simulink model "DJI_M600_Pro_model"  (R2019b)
settings: Solver=FixedStepAuto  StartTime=0.0  StopTime=stop_time  FixedStep=ts_hexacopter  RelTol=1e-3
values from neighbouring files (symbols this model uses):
  Alt_den = [0.1 1 0]    [Model_3D_init.m]
  Alt_err = 0.3817    [Model_3D_init.m]
  Alt_num = -[2 1]*18    [Model_3D_init.m]
  DvD = -5    [Model_3D_init.m]
  DvN = -17    [Model_3D_init.m]
  DvT = -17    [Model_3D_init.m]
  flightctrl_flag = bin2dec([HorizontalLogic; VerticalLogic; YawLogic; HorizontalCoordinate; StableMode]')    [User_defined_3D_init_run.m]
  Pden = [0.01 1]    [Model_3D_init.m]
  PI = -0.03    [Model_3D_init.m]
  pitch_max = 25/180*pi    (= 0.436332312999)    [Model_3D_init.m]
  Pnum = 100*[0.25 5]    [Model_3D_init.m]
  PP = -0.07    [Model_3D_init.m]
  r_max = 2.618    [Model_3D_init.m]
  r_min = -2.618    [Model_3D_init.m]
  Rden = [0.01 1]    [Model_3D_init.m]
  RI = 0.03    [Model_3D_init.m]
  Rnum = 100*[0.32 5]    [Model_3D_init.m]
  roll_max = 25/180*pi    (= 0.436332312999)    [Model_3D_init.m]
  RP = 0.07    [Model_3D_init.m]
  ts_hexacopter = 0.005    [Model_3D_init.m]
  UvD = 5    [Model_3D_init.m]
  UvN = 17    [Model_3D_init.m]
  UvT = 17    [Model_3D_init.m]
  Xtype = 3    [User_defined_3D_init_run.m]
  Yaw_den = [ET 1 0]    [Model_3D_init.m]
  Yaw_num = Eg*[1 Ez]    [Model_3D_init.m]
  YAWtype = 1    [User_defined_3D_init_run.m]
  Ytype = 1    [User_defined_3D_init_run.m]
  Ztype = 1    [User_defined_3D_init_run.m]
undefined symbols (not defined in the file or in its folder): DiscIntNeverNeededParam, params, Xdoublet, Xstep, YAWdoublet, YAWstep, Ydoublet, Ystep, Zdoublet, Zstep
libraries: simulink x1
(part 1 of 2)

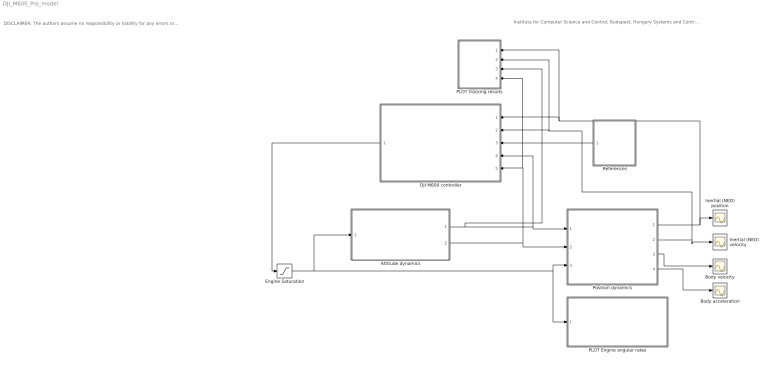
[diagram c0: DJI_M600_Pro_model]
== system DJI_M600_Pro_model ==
  note: Institute for Computer Science and Control, Budapest, Hungary Systems and Control Laboratory 2023. v3.0 12. June 2023. NED ground coordinate system and aligned (X forward, Y right, Z down) body system are applied
  note: DISCLAIMER: The authors assume no responsibility or liability for any errors or omissions in this model and any errors or damages (including loss of property or life) caused by the use of this model . The model is provided on an "as is" basis with no guarantees of fitting any specific need or goal. Application of the model in flight control design or in any application of a DJI M600 hexacopter is solely the responsibility of the user.
  Attitude dynamics : Subsystem
  Body acceleration : Scope
  Body velocity : Scope
  DJI M600 controller : Subsystem
  Engine Saturation : Saturate  UpperLimit=params.engine_saturation  LowerLimit=0
  Inertial (NED) position : Scope
  Inertial (NED) velocity : Scope
  PLOT Engine angular rates : Subsystem
  PLOT tracking results : Subsystem
  Position dynamics : Subsystem
  References : Subsystem
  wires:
  Position dynamics/1(position) -> Inertial (NED) position/1, DJI M600 controller/1(NED position), PLOT tracking results/1(NED position)
  Position dynamics/2(v_I) -> DJI M600 controller/2(NED velocity), PLOT tracking results/2(NED velocity), Inertial (NED) velocity/1
  Position dynamics/3(v_B) -> Body velocity/1
  Position dynamics/4(a_B) -> Body acceleration/1
  DJI M600 controller/1(Engine_Om_CTRL) -> Engine Saturation/1
  References/1(References) -> DJI M600 controller/3(References)
  Attitude dynamics/1(Euler angles) -> Position dynamics/1(Euler angles), DJI M600 controller/4(Euler angles), PLOT tracking results/3(Euler angles)
  Attitude dynamics/2(Omega_B) -> PLOT tracking results/4(Angular rates), DJI M600 controller/5(Angular rates), Position dynamics/2(Angular velocities)
  Engine Saturation/1 -> Attitude dynamics/1(Omega engine angualr), Position dynamics/3(Omega engine angular), PLOT Engine angular rates/1(Engine angular rates)

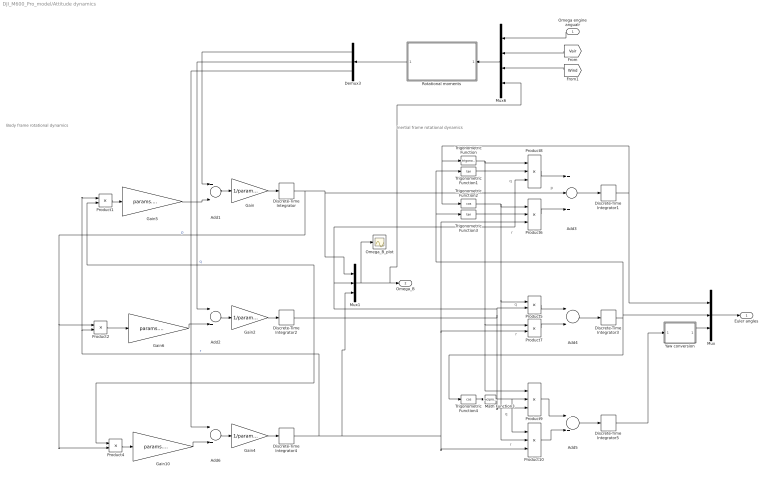
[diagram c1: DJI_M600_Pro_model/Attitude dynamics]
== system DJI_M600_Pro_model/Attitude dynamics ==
  note: r
  note: q
  note: r
  note: q
  note: r
  note: q
  note: p
  note: Inertial frame rotational dynamics
  note: Body frame rotational dynamics
  Omega engine angualr : Inport
  Add{1..2,5..6} (4 alike) : Sum
  Add3 : Sum  Inputs=+++
  Add4 : Sum  Inputs=+-
  Demux3 : Demux  Outputs=[1; 1; 1]
  Discrete-Time Integrator : DiscreteIntegrator  InitialCondition=params.initial_angvel(1)  SampleTime=ts_hexacopter  ICPrevOutput=DiscIntNeverNeededParam  ICPrevScaledInput=DiscIntNeverNeededParam
  Discrete-Time Integrator1 : DiscreteIntegrator  InitialCondition=params.initial_euler(1)  SampleTime=ts_hexacopter  ICPrevOutput=DiscIntNeverNeededParam  ICPrevScaledInput=DiscIntNeverNeededParam
  Discrete-Time Integrator2 : DiscreteIntegrator  InitialCondition=params.initial_angvel(2)  SampleTime=ts_hexacopter  ICPrevOutput=DiscIntNeverNeededParam  ICPrevScaledInput=DiscIntNeverNeededParam
  Discrete-Time Integrator3 : DiscreteIntegrator  InitialCondition=params.initial_euler(2)  SampleTime=ts_hexacopter  ICPrevOutput=DiscIntNeverNeededParam  ICPrevScaledInput=DiscIntNeverNeededParam
  Discrete-Time Integrator4 : DiscreteIntegrator  InitialCondition=params.initial_angvel(3)  SampleTime=ts_hexacopter  ICPrevOutput=DiscIntNeverNeededParam  ICPrevScaledInput=DiscIntNeverNeededParam
  Discrete-Time Integrator5 : DiscreteIntegrator  InitialCondition=params.initial_euler(3)  SampleTime=ts_hexacopter  ICPrevOutput=DiscIntNeverNeededParam  ICPrevScaledInput=DiscIntNeverNeededParam
  Gain : Gain  Gain=1/params.Jxx
  Gain10 : Gain  Gain=params.Jxx-params.Jyy
  Gain2 : Gain  Gain=1/params.Jyy
  Gain4 : Gain  Gain=1/params.Jzz
  Gain5 : Gain  Gain=params.Jyy-params.Jzz
  Gain6 : Gain  Gain=params.Jzz-params.Jxx
  Math Function3 : Math  Operator=reciprocal
  Mux : Mux  Inputs=[1; 1; 1]
  Mux1 : Mux  Inputs=[1; 1; 1]
  Mux6 : Mux  Inputs=[6; 3; 3; 3]
  Omega_B_plot : Scope
  Product{1..2,4..5,7} (5 alike) : Product
  Product{6,8..10} (4 alike) : Product  Inputs=3
  Rotational moments : MATLAB Function  TreatAsAtomicUnit=on
  Trigonometric Function : Trigonometry
  Trigonometric Function1 : Trigonometry  Operator=tan
  Trigonometric Function2 : Trigonometry  Operator=cos
  Trigonometric Function3 : Trigonometry  Operator=tan
  Trigonometric Function4 : Trigonometry  Operator=cos
  Yaw conversion : MATLAB Function  TreatAsAtomicUnit=on  SystemSampleTime=ts_hexacopter
  Euler angles : Outport
  Omega_B : Outport  Port=2
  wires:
  Gain/1 -> Discrete-Time Integrator/1
  Add1/1 -> Gain/1
  Discrete-Time Integrator/1 -> Product4/2, Product2/1, Mux1/1, Add3/2  "p"
  Discrete-Time Integrator1/1 -> Trigonometric Function2/1, Trigonometric Function/1, Mux/1
  Discrete-Time Integrator2/1 -> Product4/1, Product1/2, Product9/3, Mux1/2, Product8/3, Product5/2  "q"
  Discrete-Time Integrator3/1 -> Trigonometric Function3/1, Trigonometric Function1/1, Mux/2, Trigonometric Function4/1
  Gain2/1 -> Discrete-Time Integrator2/1
  Discrete-Time Integrator4/1 -> Product2/2, Product1/1, Mux1/3, Product10/3, Product7/2, Product6/3  "r"
  Gain4/1 -> Discrete-Time Integrator4/1
  Discrete-Time Integrator5/1 -> Yaw conversion/1(u)
  Product1/1 -> Gain5/1
  Product2/1 -> Gain6/1
  Product4/1 -> Gain10/1
  Add3/1 -> Discrete-Time Integrator1/1
  Trigonometric Function/1 -> Product9/1, Product7/1, Product8/1
  Trigonometric Function1/1 -> Product8/2
  Trigonometric Function2/1 -> Product10/2, Product5/1, Product6/1
  Trigonometric Function3/1 -> Product6/2
  Product6/1 -> Add3/3
  Product8/1 -> Add3/1
  Add4/1 -> Discrete-Time Integrator3/1
  Product5/1 -> Add4/1
  Product7/1 -> Add4/2
  Add5/1 -> Discrete-Time Integrator5/1
  Product9/1 -> Add5/1
  Product10/1 -> Add5/2
  Trigonometric Function4/1 -> Math Function3/1
  Math Function3/1 -> Product10/1, Product9/2
  Mux1/1 -> Omega_B_plot/1, Mux6/4, Omega_B/1
  Gain5/1 -> Add1/2
  Add2/1 -> Gain2/1
  Add6/1 -> Gain4/1
  Gain10/1 -> Add6/2
  Gain6/1 -> Add2/2
  Rotational moments/1(y) -> Demux3/1
  Mux6/1 -> Rotational moments/1(u)
  Demux3/1 -> Add1/1
  Demux3/2 -> Add2/1
  Demux3/3 -> Add6/1
  Omega engine angualr/1 -> Mux6/1
  [Vair] -> Mux6/2
  [Wind] -> Mux6/3
  Mux/1 -> Euler angles/1
  Yaw conversion/1(y) -> Mux/3

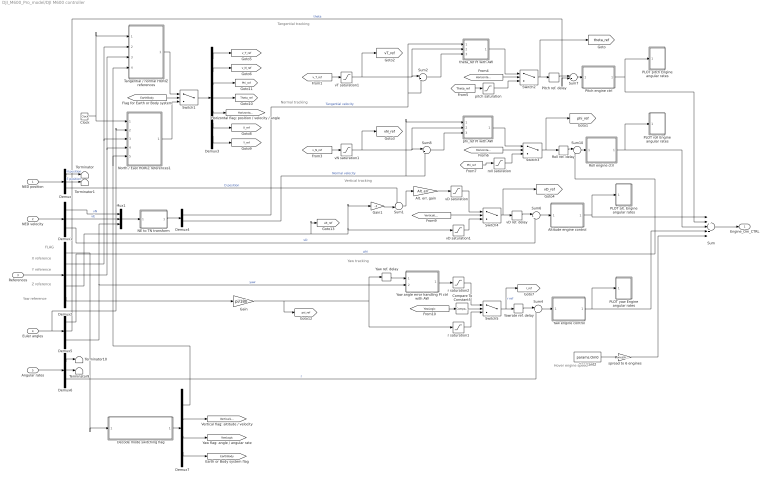
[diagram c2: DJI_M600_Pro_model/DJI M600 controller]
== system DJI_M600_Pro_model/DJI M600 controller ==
  note: Yaw reference
  note: Z reference
  note: Y reference
  note: Yaw tracking
  note: Vertical tracking
  note: Normal tracking
  note: Tangential tracking
  note: Hover engine speed
  note: FLAG
  note: X reference
  NED position : Inport
  NED velocity : Inport  Port=2
  References : Inport  Port=3
  Euler angles : Inport  Port=4
  Angular rates : Inport  Port=5
  Alt. err. gain : Gain  Gain=Alt_err
  Altitude engine control : Subsystem
  Clock : Clock
  Compare To Constant5 : simulink/Logic and Bit Operations/Compare To Constant  relop=~=  const=1  OutDataTypeStr=boolean
  Constant2 : Constant  Value=params.Om0
  Decode mode switching flag : MATLAB Function  TreatAsAtomicUnit=on  SystemSampleTime=ts_hexacopter
  Demux{,1,5..6} (4 alike) : Demux  Outputs=3
  Demux2 : Demux  Outputs=5
  Demux3 : Demux  Outputs=7
  Demux4 : Demux  Outputs=2
  Demux7 : Demux
  Gain : Gain  Gain=pi/180
  Gain1 : Gain  Gain=-1
  Mux1 : Mux  Inputs=3
  NE to TN transform : MATLAB Function  TreatAsAtomicUnit=on  SystemSampleTime=ts_hexacopter
  North / East HORIZ references1 : MATLAB Function  TreatAsAtomicUnit=on  SystemSampleTime=ts_hexacopter
  PLOT alt. Engine angular rates : Subsystem
  PLOT pitch Engine angular rates : Subsystem
  PLOT roll Engine angular rates : Subsystem
  PLOT yaw Engine angular rates : Subsystem
  Pitch engine ctrl : Subsystem
  Pitch ref. delay : Delay  DelayLength=14
  Roll engine ctrl : Subsystem
  Roll ref. delay : Delay  DelayLength=14
  Sum : Sum  Inputs=+++++
  Sum1 : Sum  Inputs=-+|
  Sum{2,4,6..8,10} (6 alike) : Sum  Inputs=|+-
  Switch1 : Switch  Criteria=u2 > Threshold
  Switch{2..5} (4 alike) : Switch  Criteria=u2 ~= 0
  Tangential / normal HORIZ references : MATLAB Function  TreatAsAtomicUnit=on  SystemSampleTime=ts_hexacopter
  Terminator{,1,9..10} (4 alike) : Terminator
  Yaw angle error handling PI ctrl with AW : MATLAB Function  TreatAsAtomicUnit=on  SystemSampleTime=ts_hexacopter
  Yaw engine control : Subsystem
  Yaw ref. delay : Delay  DelayLength=8
  Yawrate ref. delay : Delay  DelayLength=4
  phi_ref PI with AW : MATLAB Function  TreatAsAtomicUnit=on  SystemSampleTime=ts_hexacopter
  pitch saturation : Saturate  UpperLimit=pitch_max  LowerLimit=-pitch_max
  r saturation1 : Saturate  UpperLimit=r_max  LowerLimit=r_min
  r saturation2 : Saturate  UpperLimit=r_max  LowerLimit=r_min
  roll saturation : Saturate  UpperLimit=roll_max  LowerLimit=-roll_max
  spread to 6 engines : Gain  Gain=ones(6,1)
  theta_ref PI with AW : MATLAB Function  TreatAsAtomicUnit=on  SystemSampleTime=ts_hexacopter
  vD ref. delay : Delay  DelayLength=14
  vD saturation : Saturate  UpperLimit=UvD  LowerLimit=DvD
  vD saturation1 : Saturate  UpperLimit=UvD  LowerLimit=DvD
  vN saturation1 : Saturate  UpperLimit=UvN  LowerLimit=DvN
  vT saturation1 : Saturate  UpperLimit=UvT  LowerLimit=DvT
  Engine_Om_CTRL : Outport
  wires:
  Sum/1 -> Engine_Om_CTRL/1
  Altitude engine control/1(OmA) -> Sum/1, PLOT alt. Engine angular rates/1(In1)
  Sum6/1 -> Altitude engine control/1(Alt. error)
  Alt. err. gain/1 -> vD saturation/1
  Sum1/1 -> Alt. err. gain/1
  Roll engine ctrl/1(OmR) -> Sum/3, PLOT roll Engine angular rates/1(In1)
  NED position/1 -> Demux/1
  Demux/3 -> Sum1/1  "D position"
  NED velocity/1 -> Demux1/1
  References/1 -> Demux2/1
  Demux1/3 -> Sum6/2  "vD"
  Switch4/1 -> [vD_ref], vD ref. delay/1
  Demux2/4 -> [alt_ref], Gain1/1, vD saturation1/1
  Demux1/1 -> Mux1/1  "vN"
  Demux1/2 -> Mux1/2  "vE"
  Mux1/1 -> NE to TN transform/1(u)
  NE to TN transform/1(y) -> Demux4/1
  Demux4/2 -> Sum8/2, phi_ref PI with AW/1(V)  "Normal velocity"
  Demux4/1 -> theta_ref PI with AW/1(V), Sum2/2  "Tangential velocity"
  Sum4/1 -> Yaw engine control/1(Yaw error)
  Demux5/3 -> Yaw angle error handling PI ctrl with AW/2(psi), Mux1/3  "yaw"
  Switch5/1 -> [r_ref], Yawrate ref. delay/1  "r ref"
  Euler angles/1 -> Demux5/1, North / East HORIZ references1/2(Euler)
  Angular rates/1 -> Demux6/1
  Demux6/3 -> Sum4/2  "r"
  Yaw engine control/1(OmY) -> PLOT yaw Engine angular rates/1(In1), Sum/4
  Demux5/2 -> Sum7/2  "theta"
  Demux5/1 -> Sum10/2  "phi"
  Demux6/2 -> Terminator9/1
  Demux6/1 -> Terminator10/1
  Switch2/1 -> [theta_ref], Pitch ref. delay/1
  Sum2/1 -> theta_ref PI with AW/3(DV)
  Sum7/1 -> Pitch engine ctrl/1(Pitch error)
  Pitch engine ctrl/1(OmP) -> Sum/2, PLOT pitch Engine angular rates/1(In1)
  Sum8/1 -> phi_ref PI with AW/3(DV)
  Sum10/1 -> Roll engine ctrl/1(Roll error)
  vN saturation1/1 -> [vN_ref], phi_ref PI with AW/2(V_ref), Sum8/1
  Switch3/1 -> [phi_ref], Roll ref. delay/1
  spread to 6 engines/1 -> Sum/5
  Constant2/1 -> spread to 6 engines/1
  Decode mode switching flag/1(switch_signals) -> Demux7/1
  vT saturation1/1 -> theta_ref PI with AW/2(V_ref), Sum2/1, [vT_ref]
  Demux7/1 -> Tangential / normal HORIZ references/4(HorizLogic), North / East HORIZ references1/5(HorizLogic)
  Demux7/2 -> [VerticalLogic]
  Demux7/3 -> [YawLogic]
  [v_T_ref] -> vT saturation1/1
  [v_N_ref] -> vN saturation1/1
  theta_ref PI with AW/1(y) -> Switch2/1
  [HorizontalLogic] -> Switch2/2
  [Theta_ref] -> pitch saturation/1
  [HorizontalLogic] -> Switch3/2
  phi_ref PI with AW/1(y) -> Switch3/1
  [Phi_ref] -> roll saturation/1
  vD saturation/1 -> Switch4/1
  [VerticalLogic] -> Switch4/2
  Gain1/1 -> Sum1/2
  Compare To Constant5/1 -> Switch5/2
  [YawLogic] -> Compare To Constant5/1
  Yaw angle error handling PI ctrl with AW/1(r_ref) -> r saturation2/1
  Demux2/1 -> Decode mode switching flag/1(flag_dec)
  pitch saturation/1 -> Switch2/3
  roll saturation/1 -> Switch3/3
  vD saturation1/1 -> Switch4/3
  r saturation1/1 -> Switch5/3
  Demux7/4 -> [EarthBody]
  Pitch ref. delay/1 -> Sum7/1
  Roll ref. delay/1 -> Sum10/1
  vD ref. delay/1 -> Sum6/1
  Yawrate ref. delay/1 -> Sum4/1
  Demux2/5 -> Gain/1
  Yaw ref. delay/1 -> Yaw angle error handling PI ctrl with AW/1(psi_ref)
  r saturation2/1 -> Switch5/1
  [EarthBody] -> Switch1/2
  Demux3/3 -> [Phi_ref]
  Switch1/1 -> Demux3/1
  Demux3/1 -> [v_T_ref]
  Demux3/2 -> [v_N_ref]
  Demux3/4 -> [Theta_ref]
  Demux3/5 -> [HorizontalLogic]
  Demux2/2 -> Tangential / normal HORIZ references/2(X_ref), North / East HORIZ references1/3(X_ref)
  Demux2/3 -> Tangential / normal HORIZ references/3(Y_ref), North / East HORIZ references1/4(Y_ref)
  Clock/1 -> Tangential / normal HORIZ references/1(t), North / East HORIZ references1/1(t)
  Demux/1 -> Terminator/1  "N position"
  Demux/2 -> Terminator1/1  "E position"
  North / East HORIZ references1/1(y) -> Switch1/3
  Tangential / normal HORIZ references/1(y) -> Switch1/1
  Demux3/6 -> [X_ref]
  Demux3/7 -> [Y_ref]
  Gain/1 -> [psi_ref], Yaw ref. delay/1, r saturation1/1

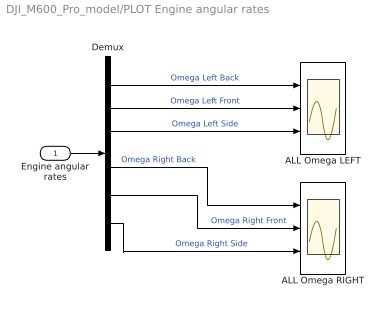
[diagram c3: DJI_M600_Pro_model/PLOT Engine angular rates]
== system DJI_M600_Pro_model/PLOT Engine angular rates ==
  Engine angular rates : Inport
  ALL Omega LEFT : Scope  NumInputPorts=3
  ALL Omega RIGHT : Scope  NumInputPorts=3
  Demux : Demux  Outputs=6
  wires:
  Demux/1 -> ALL Omega LEFT/1  "Omega Left Back"
  Engine angular rates/1 -> Demux/1
  Demux/2 -> ALL Omega LEFT/2  "Omega Left Front"
  Demux/3 -> ALL Omega LEFT/3  "Omega Left Side"
  Demux/5 -> ALL Omega RIGHT/2  "Omega Right Front"
  Demux/4 -> ALL Omega RIGHT/1  "Omega Right Back"
  Demux/6 -> ALL Omega RIGHT/3  "Omega Right Side"

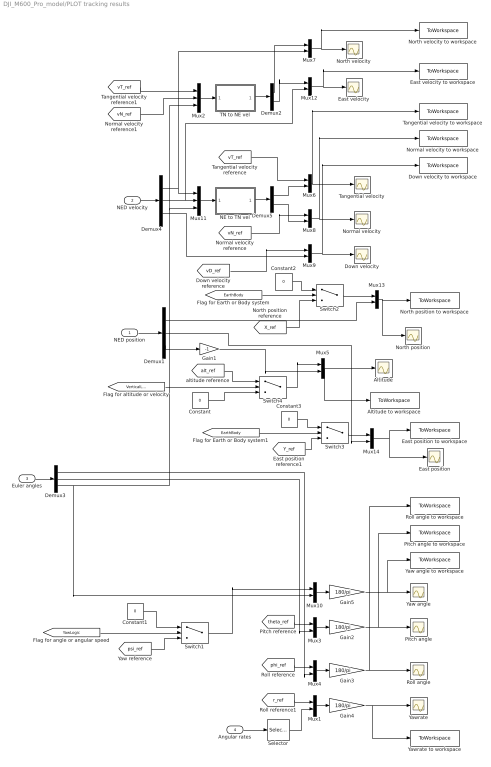
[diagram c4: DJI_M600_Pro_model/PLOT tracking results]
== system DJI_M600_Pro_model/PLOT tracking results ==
  NED position : Inport
  NED velocity : Inport  Port=2
  Euler angles : Inport  Port=3
  Angular rates : Inport  Port=4
  Altitude : Scope
  Altitude to workspace : ToWorkspace  VariableName=h  SaveFormat=Structure With Time  SampleTime=-1
  Constant{,1..3} (4 alike) : Constant  Value=0
  Demux1 : Demux  Outputs=3
  Demux2 : Demux  Outputs=2
  Demux3 : Demux  Outputs=3
  Demux4 : Demux  Outputs=3
  Demux5 : Demux  Outputs=2
  Down velocity : Scope
  Down velocity to workspace : ToWorkspace  VariableName=SvD  SaveFormat=Structure With Time  SampleTime=-1
  East position : Scope
  East position to workspace : ToWorkspace  VariableName=SE  SaveFormat=Structure With Time  SampleTime=-1
  East velocity : Scope
  East velocity to workspace : ToWorkspace  VariableName=SvEa  SaveFormat=Structure With Time  SampleTime=-1
  Gain1 : Gain  Gain=-1
  Gain{2..5} (4 alike) : Gain  Gain=180/pi
  Mux{1,3..10,12..14} (12 alike) : Mux  Inputs=2
  Mux11 : Mux  Inputs=3
  Mux2 : Mux  Inputs=3
  NE to TN vel : MATLAB Function  TreatAsAtomicUnit=on
  Normal velocity : Scope
  Normal velocity to workspace : ToWorkspace  VariableName=SvN  SaveFormat=Structure With Time  SampleTime=-1
  North position : Scope
  North position to workspace : ToWorkspace  VariableName=SN  SaveFormat=Structure With Time  SampleTime=-1
  North velocity : Scope
  North velocity to workspace : ToWorkspace  VariableName=SvNo  SaveFormat=Structure With Time  SampleTime=-1
  Pitch angle : Scope
  Pitch angle to workspace : ToWorkspace  VariableName=theta  SaveFormat=Structure With Time  SampleTime=-1
  Roll angle : Scope
  Roll angle to workspace : ToWorkspace  VariableName=phi  SaveFormat=Structure With Time  SampleTime=-1
  Selector : Selector  InputPortWidth=3  IndexOptions=Index vector (dialog)  Indices=[3]  OutputSizes=1
  Switch1 : Switch  Criteria=u2 ~= 0
  Switch2 : Switch  Criteria=u2 > Threshold
  Switch3 : Switch  Criteria=u2 > Threshold
  Switch4 : Switch  Criteria=u2 ~= 0
  TN to NE vel : MATLAB Function  TreatAsAtomicUnit=on
  Tangential velocity : Scope
  Tangential velocity to workspace : ToWorkspace  VariableName=SvT  SaveFormat=Structure With Time  SampleTime=-1
  Yaw angle : Scope
  Yaw angle to workspace : ToWorkspace  VariableName=psi  SaveFormat=Structure With Time  SampleTime=-1
  Yawrate : Scope
  Yawrate to workspace : ToWorkspace  VariableName=r  SaveFormat=Structure With Time  SampleTime=-1
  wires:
  Demux1/3 -> Gain1/1
  Mux5/1 -> Altitude to workspace/1, Altitude/1
  NED position/1 -> Demux1/1
  Euler angles/1 -> Demux3/1
  Gain5/1 -> Yaw angle to workspace/1, Yaw angle/1
  Mux10/1 -> Gain5/1
  Gain1/1 -> Mux5/2
  Demux3/3 -> Mux10/2, Mux2/3, Mux11/3
  Gain2/1 -> Pitch angle to workspace/1, Pitch angle/1
  Mux3/1 -> Gain2/1
  Gain3/1 -> Roll angle to workspace/1, Roll angle/1
  Mux4/1 -> Gain3/1
  Demux3/1 -> Mux4/2
  Demux3/2 -> Mux3/2
  [theta_ref] -> Mux3/1
  [phi_ref] -> Mux4/1
  NED velocity/1 -> Demux4/1
  Mux6/1 -> Tangential velocity to workspace/1, Tangential velocity/1
  Mux8/1 -> Normal velocity to workspace/1, Normal velocity/1
  Mux9/1 -> Down velocity to workspace/1, Down velocity/1
  Demux4/2 -> Mux12/2, Mux11/2
  Mux11/1 -> NE to TN vel/1(u)
  Demux4/1 -> Mux7/2, Mux11/1
  NE to TN vel/1(y) -> Demux5/1
  Demux4/3 -> Mux9/2
  Demux5/1 -> Mux6/2
  Demux5/2 -> Mux8/2
  [vD_ref] -> Mux9/1
  Switch1/1 -> Mux10/1
  [vN_ref] -> Mux8/1
  [VerticalLogic] -> Switch4/2
  Constant/1 -> Switch4/3
  [alt_ref] -> Switch4/1
  Switch4/1 -> Mux5/1
  [YawLogic] -> Switch1/2
  Constant1/1 -> Switch1/1
  [psi_ref] -> Switch1/3
  [vT_ref] -> Mux6/1
  [r_ref] -> Mux1/1
  Mux1/1 -> Gain4/1
  Gain4/1 -> Yawrate to workspace/1, Yawrate/1
  Selector/1 -> Mux1/2
  Angular rates/1 -> Selector/1
  Mux2/1 -> TN to NE vel/1(u)
  [vT_ref] -> Mux2/1
  [vN_ref] -> Mux2/2
  TN to NE vel/1(y) -> Demux2/1
  Demux2/1 -> Mux7/1
  Demux2/2 -> Mux12/1
  Mux7/1 -> North velocity to workspace/1, North velocity/1
  Mux12/1 -> East velocity to workspace/1, East velocity/1
  [EarthBody] -> Switch2/2
  [X_ref] -> Switch2/3
  Mux13/1 -> North position/1, North position to workspace/1
  Switch2/1 -> Mux13/1
  Demux1/1 -> Mux13/2
  Constant2/1 -> Switch2/1
  [EarthBody] -> Switch3/2
  Constant3/1 -> Switch3/1
  [Y_ref] -> Switch3/3
  Switch3/1 -> Mux14/1
  Mux14/1 -> East position/1, East position to workspace/1
  Demux1/2 -> Mux14/2

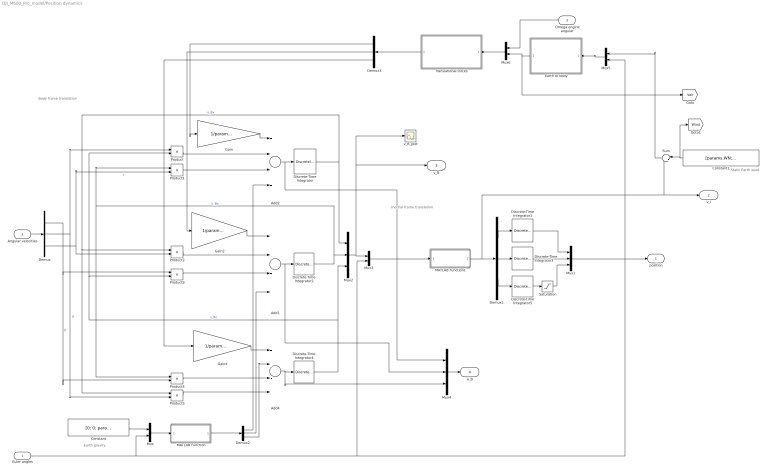
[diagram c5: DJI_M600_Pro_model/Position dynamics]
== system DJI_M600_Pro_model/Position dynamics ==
  note: Static Earth wind
  note: Earth gravity
  note: Inertial frame translation
  note: Body frame translation
  Euler angles : Inport
  Angular velocities : Inport  Port=2
  Omega engine angular : Inport  Port=3
  Add1 : Sum  Inputs=+-++
  Add2 : Sum  Inputs=+-++
  Add4 : Sum  Inputs=++-+
  Constant : Constant  Value=[0; 0; params.g]  VectorParams1D=off
  Constant1 : Constant  Value=[params.WN; params.WE; params.WD]  VectorParams1D=off
  Demux : Demux  Outputs=3
  Demux1 : Demux  Outputs=[1; 1; 1]
  Demux2 : Demux  Outputs=3
  Demux3 : Demux  Outputs=[1; 1; 1]
  Discrete-Time Integrator : DiscreteIntegrator  InitialCondition=params.initial_speed(1)  SampleTime=ts_hexacopter  ICPrevOutput=DiscIntNeverNeededParam  ICPrevScaledInput=DiscIntNeverNeededParam
  Discrete-Time Integrator1 : DiscreteIntegrator  InitialCondition=params.initial_pos(1)  SampleTime=ts_hexacopter  ICPrevOutput=DiscIntNeverNeededParam  ICPrevScaledInput=DiscIntNeverNeededParam
  Discrete-Time Integrator2 : DiscreteIntegrator  InitialCondition=params.initial_speed(2)  SampleTime=ts_hexacopter  ICPrevOutput=DiscIntNeverNeededParam  ICPrevScaledInput=DiscIntNeverNeededParam
  Discrete-Time Integrator3 : DiscreteIntegrator  InitialCondition=params.initial_pos(2)  SampleTime=ts_hexacopter  ICPrevOutput=DiscIntNeverNeededParam  ICPrevScaledInput=DiscIntNeverNeededParam
  Discrete-Time Integrator4 : DiscreteIntegrator  InitialCondition=params.initial_speed(3)  SampleTime=ts_hexacopter  ICPrevOutput=DiscIntNeverNeededParam  ICPrevScaledInput=DiscIntNeverNeededParam
  Discrete-Time Integrator5 : DiscreteIntegrator  InitialCondition=params.initial_pos(3)  SampleTime=ts_hexacopter  ICPrevOutput=DiscIntNeverNeededParam  ICPrevScaledInput=DiscIntNeverNeededParam
  Earth to body : MATLAB Function  TreatAsAtomicUnit=on  SystemSampleTime=ts_hexacopter
  Gain : Gain  Gain=1/params.m
  Gain2 : Gain  Gain=1/params.m
  Gain4 : Gain  Gain=1/params.m
  MATLAB Function : MATLAB Function  TreatAsAtomicUnit=on  SystemSampleTime=ts_hexacopter
  MATLAB Function1 : MATLAB Function  TreatAsAtomicUnit=on  SystemSampleTime=ts_hexacopter
  Mux : Mux  Inputs=[3; 3]
  Mux1 : Mux  Inputs=[1; 1; 1]
  Mux2 : Mux  Inputs=[1; 1; 1]
  Mux3 : Mux  Inputs=[3; 3]
  Mux4 : Mux  Inputs=[1; 1; 1]
  Mux5 : Mux  Inputs=[3; 3]
  Mux6 : Mux  Inputs=[6; 3]
  Product{,1..5} (6 alike) : Product
  Saturation : Saturate  UpperLimit=0  LowerLimit=-inf
  Sum : Sum  Inputs=|-+
  Translational forces : MATLAB Function  TreatAsAtomicUnit=on  SystemSampleTime=ts_hexacopter
  v_B_plot : Scope
  position : Outport
  v_I : Outport  Port=2
  v_B : Outport  Port=3
  a_B : Outport  Port=4
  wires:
  Discrete-Time Integrator/1 -> Product5/1, Product2/1, Mux2/1  "v_Bx"
  Discrete-Time Integrator1/1 -> Mux1/1
  Discrete-Time Integrator2/1 -> Product4/1, Product1/1, Mux2/2  "v_By"
  Discrete-Time Integrator3/1 -> Mux1/2
  Discrete-Time Integrator4/1 -> Mux2/3, Product3/2, Product/2  "v_Bz"
  Discrete-Time Integrator5/1 -> Saturation/1
  Add4/1 -> Mux4/3, Discrete-Time Integrator4/1
  Gain4/1 -> Add4/1
  Demux3/3 -> Gain4/1
  MATLAB Function1/1(v_I) -> v_I/1, Sum/2, Demux1/1
  Saturation/1 -> Mux1/3
  Angular velocities/1 -> Demux/1
  Demux3/1 -> Gain/1
  Gain/1 -> Add2/1
  Add2/1 -> Mux4/1, Discrete-Time Integrator/1
  Product/1 -> Add2/2
  Demux/2 -> Product/1, Product5/2  "q"
  Product1/1 -> Add2/3
  Demux/3 -> Product1/2, Product2/2  "r"
  Gain2/1 -> Add1/1
  Add1/1 -> Mux4/2, Discrete-Time Integrator2/1
  Product3/1 -> Add1/3
  Product2/1 -> Add1/2
  Demux/1 -> Product4/2, Product3/1  "p"
  Product5/1 -> Add4/4
  Product4/1 -> Add4/3
  Euler angles/1 -> Mux5/2, Mux3/2, Mux/2
  Mux3/1 -> MATLAB Function1/1(u)
  Demux1/1 -> Discrete-Time Integrator1/1
  Demux1/2 -> Discrete-Time Integrator3/1
  Demux1/3 -> Discrete-Time Integrator5/1
  Constant/1 -> Mux/1
  Mux/1 -> MATLAB Function/1(u)
  MATLAB Function/1(y_B) -> Demux2/1
  Demux2/3 -> Add4/2
  Demux2/2 -> Add1/4
  Demux2/1 -> Add2/4
  Mux2/1 -> v_B_plot/1, v_B/1, Mux3/1
  Mux4/1 -> a_B/1
  Constant1/1 -> [Wind], Sum/1
  Mux5/1 -> Earth to body/1(u)
  Sum/1 -> Mux5/1
  Mux6/1 -> Translational forces/1(u)
  Earth to body/1(y_B) -> [Vair], Mux6/2
  Omega engine angular/1 -> Mux6/1
  Translational forces/1(y) -> Demux3/1
  Demux3/2 -> Gain2/1
  Mux1/1 -> position/1

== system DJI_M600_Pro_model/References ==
  User defined references : Subsystem
  References : Outport
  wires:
  User defined references/1(User references) -> References/1

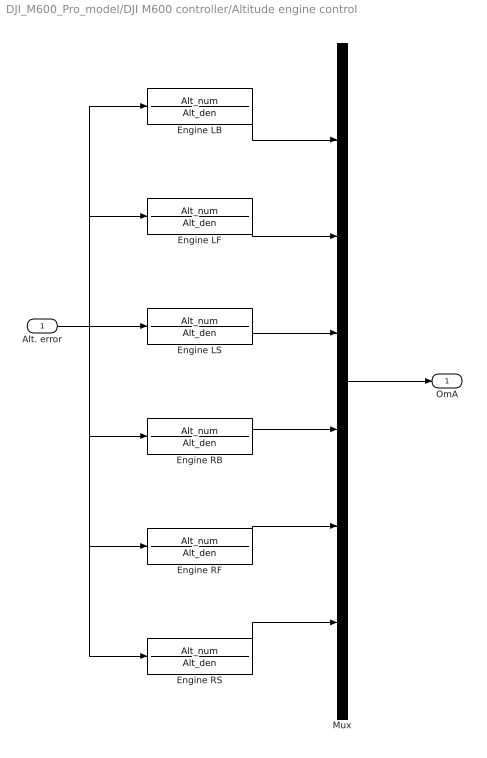
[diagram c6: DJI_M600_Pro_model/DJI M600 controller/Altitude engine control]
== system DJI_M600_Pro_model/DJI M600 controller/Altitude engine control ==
  Alt. error : Inport
  Engine LB : TransferFcn  Numerator=Alt_num  Denominator=Alt_den
  Engine LF : TransferFcn  Numerator=Alt_num  Denominator=Alt_den
  Engine LS : TransferFcn  Numerator=Alt_num  Denominator=Alt_den
  Engine RB : TransferFcn  Numerator=Alt_num  Denominator=Alt_den
  Engine RF : TransferFcn  Numerator=Alt_num  Denominator=Alt_den
  Engine RS : TransferFcn  Numerator=Alt_num  Denominator=Alt_den
  Mux : Mux  Inputs=6
  OmA : Outport
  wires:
  Alt. error/1 -> Engine LS/1, Engine LF/1, Engine LB/1, Engine RB/1, Engine RF/1, Engine RS/1
  Mux/1 -> OmA/1
  Engine LB/1 -> Mux/1
  Engine LF/1 -> Mux/2
  Engine LS/1 -> Mux/3
  Engine RB/1 -> Mux/4
  Engine RF/1 -> Mux/5
  Engine RS/1 -> Mux/6

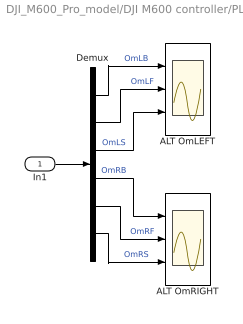
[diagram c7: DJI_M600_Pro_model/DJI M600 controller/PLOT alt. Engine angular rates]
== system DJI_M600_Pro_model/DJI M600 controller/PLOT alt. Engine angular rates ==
  In1 : Inport
  ALT OmLEFT : Scope  NumInputPorts=3
  ALT OmRIGHT : Scope  NumInputPorts=3
  Demux : Demux  Outputs=6
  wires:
  Demux/1 -> ALT OmLEFT/1  "OmLB"
  In1/1 -> Demux/1
  Demux/2 -> ALT OmLEFT/2  "OmLF"
  Demux/3 -> ALT OmLEFT/3  "OmLS"
  Demux/5 -> ALT OmRIGHT/2  "OmRF"
  Demux/4 -> ALT OmRIGHT/1  "OmRB"
  Demux/6 -> ALT OmRIGHT/3  "OmRS"

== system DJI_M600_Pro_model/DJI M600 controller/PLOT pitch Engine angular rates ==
  In1 : Inport
  Demux : Demux  Outputs=6
  Pitch OmLEFT : Scope  NumInputPorts=3
  Pitch OmRIGHT : Scope  NumInputPorts=3
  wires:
  Demux/1 -> Pitch OmLEFT/1  "OmLB"
  In1/1 -> Demux/1
  Demux/2 -> Pitch OmLEFT/2  "OmLF"
  Demux/3 -> Pitch OmLEFT/3  "OmLS"
  Demux/5 -> Pitch OmRIGHT/2  "OmRF"
  Demux/4 -> Pitch OmRIGHT/1  "OmRB"
  Demux/6 -> Pitch OmRIGHT/3  "OmRS"

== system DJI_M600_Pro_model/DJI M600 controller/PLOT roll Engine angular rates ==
  In1 : Inport
  Demux : Demux  Outputs=6
  Roll OmLEFT : Scope  NumInputPorts=3
  Roll OmRIGHT : Scope  NumInputPorts=3
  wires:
  Demux/1 -> Roll OmLEFT/1  "OmLB"
  In1/1 -> Demux/1
  Demux/2 -> Roll OmLEFT/2  "OmLF"
  Demux/3 -> Roll OmLEFT/3  "OmLS"
  Demux/5 -> Roll OmRIGHT/2  "OmRF"
  Demux/4 -> Roll OmRIGHT/1  "OmRB"
  Demux/6 -> Roll OmRIGHT/3  "OmRS"

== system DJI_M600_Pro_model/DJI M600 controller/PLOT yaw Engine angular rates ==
  In1 : Inport
  Demux : Demux  Outputs=6
  YAW OmLEFT : Scope  NumInputPorts=3
  YAW OmRIGHT : Scope  NumInputPorts=3
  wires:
  Demux/1 -> YAW OmLEFT/1  "OmLB"
  In1/1 -> Demux/1
  Demux/2 -> YAW OmLEFT/2  "OmLF"
  Demux/3 -> YAW OmLEFT/3  "OmLS"
  Demux/5 -> YAW OmRIGHT/2  "OmRF"
  Demux/4 -> YAW OmRIGHT/1  "OmRB"
  Demux/6 -> YAW OmRIGHT/3  "OmRS"

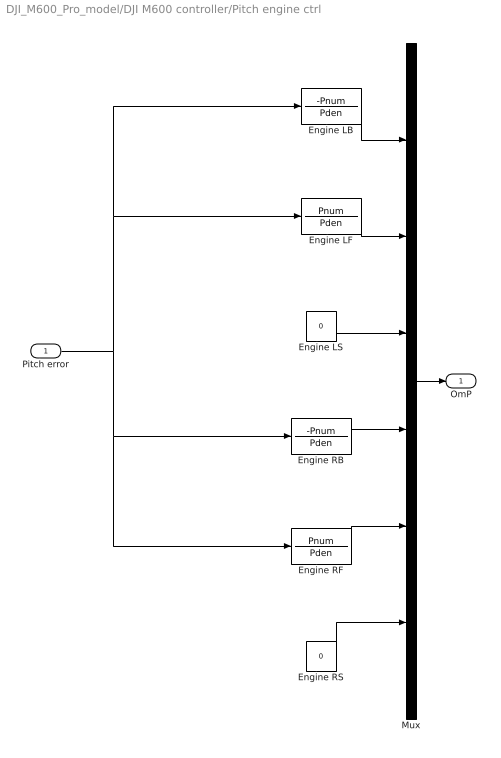
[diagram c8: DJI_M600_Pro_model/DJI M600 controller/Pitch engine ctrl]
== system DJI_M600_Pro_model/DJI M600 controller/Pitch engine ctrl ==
  Pitch error : Inport
  Engine LB : TransferFcn  Numerator=-Pnum  Denominator=Pden
  Engine LF : TransferFcn  Numerator=Pnum  Denominator=Pden
  Engine LS : Constant  Value=0
  Engine RB : TransferFcn  Numerator=-Pnum  Denominator=Pden
  Engine RF : TransferFcn  Numerator=Pnum  Denominator=Pden
  Engine RS : Constant  Value=0
  Mux : Mux  Inputs=6
  OmP : Outport
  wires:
  Pitch error/1 -> Engine LF/1, Engine LB/1, Engine RF/1, Engine RB/1
  Mux/1 -> OmP/1
  Engine RS/1 -> Mux/6
  Engine LB/1 -> Mux/1
  Engine LF/1 -> Mux/2
  Engine RB/1 -> Mux/4
  Engine RF/1 -> Mux/5
  Engine LS/1 -> Mux/3

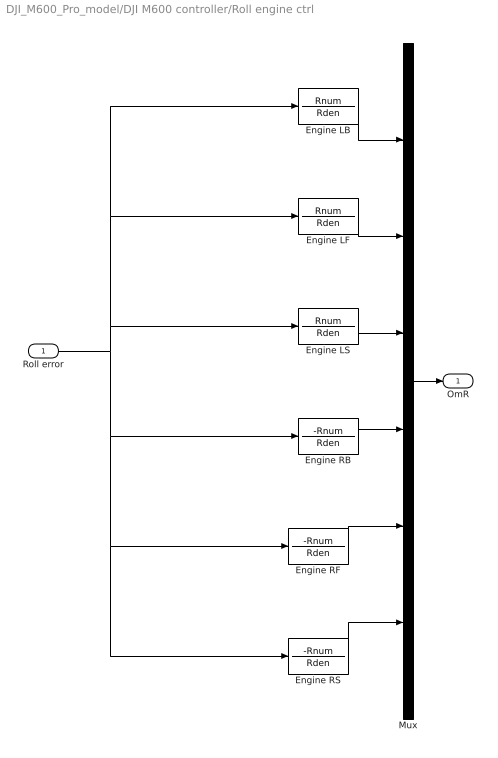
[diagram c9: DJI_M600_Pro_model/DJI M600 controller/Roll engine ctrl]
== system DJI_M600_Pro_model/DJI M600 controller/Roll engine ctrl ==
  Roll error : Inport
  Engine LB : TransferFcn  Numerator=Rnum  Denominator=Rden
  Engine LF : TransferFcn  Numerator=Rnum  Denominator=Rden
  Engine LS : TransferFcn  Numerator=Rnum  Denominator=Rden
  Engine RB : TransferFcn  Numerator=-Rnum  Denominator=Rden
  Engine RF : TransferFcn  Numerator=-Rnum  Denominator=Rden
  Engine RS : TransferFcn  Numerator=-Rnum  Denominator=Rden
  Mux : Mux  Inputs=6
  OmR : Outport
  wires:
  Roll error/1 -> Engine LF/1, Engine LB/1, Engine LS/1, Engine RS/1, Engine RF/1, Engine RB/1
  Mux/1 -> OmR/1
  Engine RS/1 -> Mux/6
  Engine LB/1 -> Mux/1
  Engine LF/1 -> Mux/2
  Engine RB/1 -> Mux/4
  Engine RF/1 -> Mux/5
  Engine LS/1 -> Mux/3

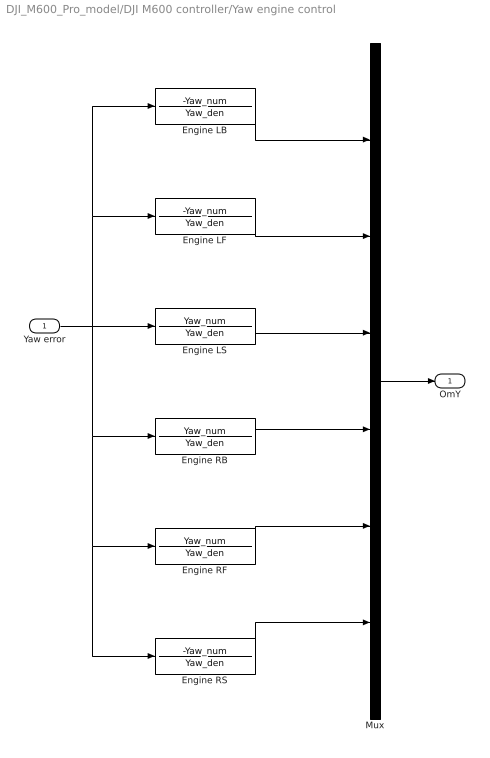
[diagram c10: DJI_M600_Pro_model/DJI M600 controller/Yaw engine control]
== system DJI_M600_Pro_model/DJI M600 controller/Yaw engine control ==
  Yaw error : Inport
  Engine LB : TransferFcn  Numerator=-Yaw_num  Denominator=Yaw_den
  Engine LF : TransferFcn  Numerator=-Yaw_num  Denominator=Yaw_den
  Engine LS : TransferFcn  Numerator=Yaw_num  Denominator=Yaw_den
  Engine RB : TransferFcn  Numerator=Yaw_num  Denominator=Yaw_den
  Engine RF : TransferFcn  Numerator=Yaw_num  Denominator=Yaw_den
  Engine RS : TransferFcn  Numerator=-Yaw_num  Denominator=Yaw_den
  Mux : Mux  Inputs=6
  OmY : Outport
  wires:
  Yaw error/1 -> Engine LS/1, Engine LF/1, Engine LB/1, Engine RB/1, Engine RF/1, Engine RS/1
  Mux/1 -> OmY/1
  Engine LB/1 -> Mux/1
  Engine LF/1 -> Mux/2
  Engine LS/1 -> Mux/3
  Engine RB/1 -> Mux/4
  Engine RF/1 -> Mux/5
  Engine RS/1 -> Mux/6

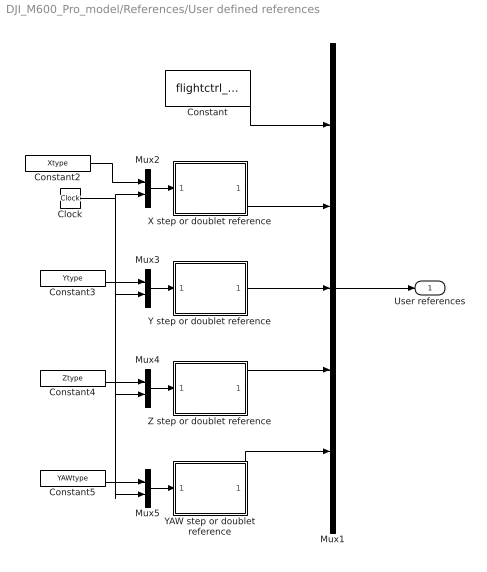
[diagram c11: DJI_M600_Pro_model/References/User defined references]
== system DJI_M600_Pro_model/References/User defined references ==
  Clock : Clock
  Constant : Constant  Value=flightctrl_flag
  Constant2 : Constant  Value=Xtype
  Constant3 : Constant  Value=Ytype
  Constant4 : Constant  Value=Ztype
  Constant5 : Constant  Value=YAWtype
  Mux1 : Mux  Inputs=5
  Mux{2..5} (4 alike) : Mux  Inputs=2
  X step or doublet reference : MATLAB Function  TreatAsAtomicUnit=on  SystemSampleTime=ts_hexacopter
  Y step or doublet reference : MATLAB Function  TreatAsAtomicUnit=on  SystemSampleTime=ts_hexacopter
  YAW step or doublet reference : MATLAB Function  TreatAsAtomicUnit=on  SystemSampleTime=ts_hexacopter
  Z step or doublet reference : MATLAB Function  TreatAsAtomicUnit=on  SystemSampleTime=ts_hexacopter
  User references : Outport
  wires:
  Constant5/1 -> Mux5/1
  Y step or doublet reference/1(y) -> Mux1/3
  Clock/1 -> Mux5/2, Mux4/2, Mux3/2, Mux2/2
  Mux3/1 -> Y step or doublet reference/1(u)
  Mux2/1 -> X step or doublet reference/1(u)
  YAW step or doublet reference/1(y) -> Mux1/5
  Constant2/1 -> Mux2/1
  Mux5/1 -> YAW step or doublet reference/1(u)
  X step or doublet reference/1(y) -> Mux1/2
  Constant4/1 -> Mux4/1
  Mux4/1 -> Z step or doublet reference/1(u)
  Z step or doublet reference/1(y) -> Mux1/4
  Mux1/1 -> User references/1
  Constant/1 -> Mux1/1
  Constant3/1 -> Mux3/1

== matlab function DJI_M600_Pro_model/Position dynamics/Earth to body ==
function y_B = inertialtobody(u)
% Transformation of input Earth airspeed into body airspeed
% Inputs:
% u(1:3):   Inertial airspeed [m/s]
% u(4:6):   roll, pitch, yaw Euler angles [rad]
%
% Institute for Computer Science and Control,  Budapest, Hungary
% Systems and Control Laboratory 2023.
% v3.0 12. June 2023.
%

% Separate inputs
% Inertial airspeed
u_I = u(1:3);
% Euler angles
phi = u(4);
theta = u(5);
psi = u(6);

% Create inertial to body rotation matrix
R_1 = [1 0 0; 0 cos(phi) sin(phi); 0 -sin(phi) cos(phi)];
R_2 = [cos(theta) 0 -sin(theta); 0 1 0; sin(theta) 0 cos(theta)];
R_3 = [cos(psi) sin(psi) 0; -sin(psi) cos(psi) 0; 0 0 1];

R_BI = R_1*R_2*R_3;

% Output is body airspeed
y_B = R_BI*u_I;

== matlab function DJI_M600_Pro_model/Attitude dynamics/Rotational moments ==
function y = fcn(u,params)
% Function to calculate the rotational moments around the axes of the body
% system
% Inputs:
% u(1)-u(6):    rotor angular rates [rad/s]
% u(7)-u(9):    Airspeed in body system [m/s]
% u(10)-u(12):  Windspeed in Earth system [m/s]
% u(13)-u(15):  body angular rates [rad/s]
% Outputs:
% Tx X body torque [Nm]
% Ty Y body torque [Nm]
% Tz Z body torque [Nm]
%
% Institute for Computer Science and Control,  Budapest, Hungary
% Systems and Control Laboratory 2023.
% v3.0 12. June 2023.
%

% Vertical airspeed component:
Vaz=u(9);

% Vertical gain:
Kc=0.0243*Vaz^2+2.8851;

% Air geometric constant
cAG=params.rho*params.A*params.R;

% Body Z torque
Tz=-params.Kr*u(15).*abs(u(15))+params.cP0/100*cAG*params.R^2*(-u(1).^2-u(2).^2+u(3).^2+u(4).^2+u(5).^2-u(6).^2);

% Body X torque
Tx=-u(14)*params.Jr*(u(1)+u(2)-u(3)-u(4)-u(5)+u(6))+...
    params.cT0*cAG*params.R/2*params.l*(u(1)^2+u(2)^2+2*u(3)^2-u(4)^2-u(5)^2-2*u(6)^2)+...          
     Kc/100*cAG*params.l/2*Vaz*(u(1)+u(2)+2*u(3)-u(4)-u(5)-2*u(6))-10*u(13)*abs(u(13));

% Body Y torque
Ty=u(13)*params.Jr*(u(1)+u(2)-u(3)-u(4)-u(5)+u(6))+...
    params.cT0*cAG*params.R*sqrt(3)/2*params.l*(-u(1)^2+u(2)^2-u(4)^2+u(5)^2)+...          
     Kc/100*cAG*sqrt(3)*params.l/2*Vaz*(-u(1)+u(2)-u(4)+u(5))-10*u(14)*abs(u(14));

% Function output
y = [Tx; Ty; Tz];

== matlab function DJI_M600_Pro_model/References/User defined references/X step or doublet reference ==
function y = fcn(u, Xstep, Xdoublet)
% X direction reference signal generation
% Inputs:
% u(1): type of required reference
% u(2): absolute time [s]
% Parameters:
% Xstep:    parameter structure of step (type 1) reference
% Xdoublet: parameter  structures of doublet (type 2), half doublet (type 3) and
%           elonged doublet (type 4) references
% For details see: User_defined_3D_init_run.m script
%
% Institute for Computer Science and Control,  Budapest, Hungary
% Systems and Control Laboratory 2023.
% v3.0 12. June 2023.
% 


    persistent start    
    % Save parameter structures into local values:
    step=Xstep;
    doublet=Xdoublet;
    
    % Initialize persistent variable upon startup
    if isempty(start)
        start = 0;
    end
    
    % Save time of start
    if (start==0)
        start = u(2);
    end
    
    % Default value for case of undefined parameters:
    ref=0;
    
    switch u(1)
        case 1 % step reference required
            if (u(2)<start + step.step) % Output before step
                ref=step.zero;
            else                        % Output after step
                ref=step.zero + step.amp;
            end   
            
        case 2 % doublet reference required
            if (u(2)<start + doublet.step) % Output before doublet
                ref=doublet.zero;
            elseif (u(2)>=(start + doublet.step) && u(2)<(start + doublet.step + doublet.period/2)) % First, positive period
                ref=doublet.zero + doublet.amp;
            elseif (u(2)>=(start + doublet.step + doublet.period/2) && u(2)<(start + doublet.step + doublet.period)) % Second, negative period
                ref=doublet.zero- doublet.amp;
            else                            % Output after doublet
                ref=doublet.zero;
            end                    
        case 3 % half doublet reference required
            if (u(2)<start + doublet.step) % Output before half doublet
                ref=doublet.zero;
            elseif (u(2)>=(start + doublet.step) && u(2)<(start + doublet.step + doublet.period)) % Half doublet output (positive)
                ref=doublet.zero + doublet.amp;            
            else                           % Output after half doublet
                ref=doublet.zero; 
            end   
        case 4 % elongated doublet reference required (1.5 period long with gap)
            if (u(2)<start + doublet.step)      % Output before elongated doublet
                ref=doublet.zero;
            elseif (u(2)>=(start + doublet.step) && u(2)<(start + doublet.step + doublet.period/2)) % First, positive period
                ref=doublet.zero + doublet.amp;
            elseif (u(2)>=(start + doublet.step + doublet.period/2) && u(2)<(start + doublet.step + doublet.period)) % Gap with zero level output
                ref=doublet.zero;
            elseif (u(2)>=(start + doublet.step + doublet.period) && u(2)<(start + doublet.step + 3*doublet.period/2)) % Second, negative period
                ref=doublet.zero - doublet.amp;
            else                                % Output after elongated doublet
                ref=doublet.zero;
            end
    end
    
    y = ref; % Function output (actual value of reference)
end

== matlab function DJI_M600_Pro_model/DJI M600 controller/North // East 
HORIZ references1 ==
function y  = NEcntrl(t,Euler,X_ref,Y_ref,HorizLogic)
% Processing of references for control in North / East
% directions (converted into body system of M600)
% Inputs:
% t:            time [s]
% Euler(3):     Euler angles [phi, theta, psi]
% X_ref:        X reference
% Y_ref:        Y reference
% HorizLogic:   horizontal logic flag
% Outputs:
% v_T_ref:      Tangential velocity reference
% v_N_ref:      Normal velocity reference
% Phi_ref:      Roll reference
% Theta_ref:    Theta reference
% HLogic:       the same flight mode flag as the input, or a modified one
%               when returning from angle track to braking mode with zero
%               velocity
% X_ref:        X position reference (North / Tangential)
% Y_ref:        Y position reference (East / Normal)
%
% Institute for Computer Science and Control,  Budapest, Hungary
% Systems and Control Laboratory 2023.
% v3.0 12. June 2023.
% 

% Persistent variables:
% Init flag of Position kick control
persistent Pinit
% Start time of position kick control
persistent t0
% X and Y reference amplitudes to be applied
% (not necessarily the same as X_ref and Y_ref)
persistent Xamp
persistent Yamp
% Flag for Position step mode
persistent Pstep

% Initialize permanent variables upon startup
if isempty(Pinit)
    Pinit=0;
    t0=0;
    Xamp=0;
    Yamp=0;
    Pstep=0;
end

% Switch horizontal logic flag
switch HorizLogic
    case 0 % Angle references
        if (X_ref~=0 || Y_ref~=0)  % Normal angle tracking (convert deg to rad)      
            % Transformation with North / East angles:
            % Reference angles and measured heading converted to rad
            aN=X_ref/180*pi;
            aE=Y_ref/180*pi;
            psi=Euler(3);
            % Construct transformation from rotated body system to NED
            Tp=[cos(psi) -sin(psi) 0; sin(psi) cos(psi) 0; 0 0 1];
            TN=[1 0 0; 0 cos(aN) -sin(aN); 0 sin(aN) cos(aN)];
            TE=[cos(aE) 0 sin(aE); 0 1 0; -sin(aE) 0 cos(aE)];
            M=TE*TN*Tp;
            % Obtain Euler angles from the transformation
            vEu=rotm2eul(M);            
            y=[0; 0; vEu(3); vEu(2); 0; 0; 0];
        elseif (X_ref==0 && Y_ref==0) % Change to velocity track for braking
            y=[0; 0; 0; 0; 1; 0; 0];
        else % Safe output with zero references
            y=[0; 0; 0; 0; 1; 0; 0];
        end
    case 1 % Velocity references
        % Transform X and Y references (North / east) to tangential and normal velocities
        psi=Euler(3);
        y=[cos(psi)*X_ref+sin(psi)*Y_ref; -sin(psi)*X_ref+cos(psi)*Y_ref; 0; 0; 1; 0; 0];
    case 2 % Position references
        if (X_ref~=0 || Y_ref~=0 || 1==Pinit) % Nonzero references start kick control
            if (0==Pinit)
                Pinit=1;
                t0=t;
                Xamp=X_ref;
                Yamp=Y_ref;
            end
            if (t-t0<=0.75 && 0==Pstep) % Not real position, limited time velocity reference is given (kick control)
                if (t-t0>0.5 && (X_ref~=0 || Y_ref~=0)) % Switch to step reference mode if long reference comes
                    Pstep=1;
                end
                % Transform North / East velocity references to tangential and normal
                psi=Euler(3);
                y=[cos(psi)*Xamp+sin(psi)*Yamp; -sin(psi)*Xamp+cos(psi)*Yamp; 0; 0; 1; X_ref; Y_ref];
            elseif (1==Pstep) % Position step mode with long reference
                Xamp=sign(X_ref)*min([abs(X_ref)/2,3]);
                Yamp=sign(Y_ref)*min([abs(Y_ref)/2,3]);
                % Transform North / East velocity references to tangential and normal
                psi=Euler(3);
                y=[cos(psi)*Xamp+sin(psi)*Yamp; -sin(psi)*Xamp+cos(psi)*Yamp; 0; 0; 1; X_ref; Y_ref];
                % Switch back from position step mode if references are
                % again zero
                if (0==X_ref && 0==Y_ref)
                    Pstep=0;
                end
            else % Safe output with zero references, and re-init position kick mode
                y=[0; 0; 0; 0; 1; 0; 0];
                Pinit=0;
            end
        else % Safe output with zero references
            y=[0; 0; 0; 0; 1; 0; 0];
        end            
    otherwise   % Safe mode with velocity flag and zero velocity references
        y=[0; 0; 0; 0; 1; 0; 0];
end

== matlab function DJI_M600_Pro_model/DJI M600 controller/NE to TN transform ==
function y = fcn(u)
% Transform North-East to Tangential-Normal (body X-Y) directions
% Inputs
% u(1):     North position / velocity
% u(2):     East position / velocity
% u(3):     real Yaw angle
% Outputs
% T:    tangential position / velocity
% N:    normal position / velocity
%
% Institute for Computer Science and Control,  Budapest, Hungary
% Systems and Control Laboratory 2023.
% v3.0 12. June 2023.
%   

y = [u(1)*cos(u(3))+u(2)*sin(u(3)); -u(1)*sin(u(3))+u(2)*cos(u(3))];

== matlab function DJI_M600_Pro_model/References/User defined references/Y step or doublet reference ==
function y = fcn(u, Ystep, Ydoublet)
% Y direction reference signal generation
% Inputs:
% u(1): type of required reference
% u(2): absolute time [s]
% Parameters:
% Ystep:    parameter structure of step (type 1) reference
% Ydoublet: parameter  structures of doublet (type 2), half doublet (type 3) and
%           elonged doublet (type 4) references
% For details see: User_defined_3D_init_run.m script
%
% Institute for Computer Science and Control,  Budapest, Hungary
% Systems and Control Laboratory 2023.
% v3.0 12. June 2023.
% 


    persistent start    
    % Save parameter structures into local values:
    step=Ystep;
    doublet=Ydoublet;
    
    % Initialize persistent variable upon startup
    if isempty(start)
        start = 0;
    end
    
    % Save time of start
    if (start==0)
        start = u(2);
    end
    
    % Default value for case of undefined parameters:
    ref=0;
    
    switch u(1)
        case 1 % step reference required
            if (u(2)<start + step.step) % Output before step
                ref=step.zero;
            else                        % Output after step
                ref=step.zero + step.amp;
            end   
            
        case 2 % doublet reference required
            if (u(2)<start + doublet.step) % Output before doublet
                ref=doublet.zero;
            elseif (u(2)>=(start + doublet.step) && u(2)<(start + doublet.step + doublet.period/2)) % First, positive period
                ref=doublet.zero + doublet.amp;
            elseif (u(2)>=(start + doublet.step + doublet.period/2) && u(2)<(start + doublet.step + doublet.period)) % Second, negative period
                ref=doublet.zero- doublet.amp;
            else                            % Output after doublet
                ref=doublet.zero;
            end                    
        case 3 % half doublet reference required
            if (u(2)<start + doublet.step) % Output before half doublet
                ref=doublet.zero;
            elseif (u(2)>=(start + doublet.step) && u(2)<(start + doublet.step + doublet.period)) % Half doublet output (positive)
                ref=doublet.zero + doublet.amp;            
            else                           % Output after half doublet
                ref=doublet.zero; 
            end   
        case 4 % elongated doublet reference required (1.5 period long with gap)
            if (u(2)<start + doublet.step)      % Output before elongated doublet
                ref=doublet.zero;
            elseif (u(2)>=(start + doublet.step) && u(2)<(start + doublet.step + doublet.period/2)) % First, positive period
                ref=doublet.zero + doublet.amp;
            elseif (u(2)>=(start + doublet.step + doublet.period/2) && u(2)<(start + doublet.step + doublet.period)) % Gap with zero level output
                ref=doublet.zero;
            elseif (u(2)>=(start + doublet.step + doublet.period) && u(2)<(start + doublet.step + 3*doublet.period/2)) % Second, negative period
                ref=doublet.zero - doublet.amp;
            else                                % Output after elongated doublet
                ref=doublet.zero;
            end
    end
    
    y = ref; % Function output (actual value of reference)
end

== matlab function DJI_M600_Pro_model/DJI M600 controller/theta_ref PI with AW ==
function y = fcn(V,V_ref,DV,PP,PI,ts_hexacopter,pitch_max)
% PI control of pitch angle with anti-windup (AW)
% Inputs:
% V:    actual velocity value
% DV:   velocity tracking error
% Parameters:
% PP:               pitch proportional gain
% PI:               pitch integral gain
% ts_hexacopter:    sampling time
% pitch_max:        maximum allowed pitch angle
% Output:
% dmd:  pitch angle reference
%
% Institute for Computer Science and Control,  Budapest, Hungary
% Systems and Control Laboratory 2023.
% v3.0 12. June 2023.
%

% State of integral control
persistent state
% PP gain scale in brake mode
persistent scPP

% Initialize persistent variables
if isempty(state)
    state = 0;
    % By default no brake scale
    scPP=1;
end

if (abs(DV)>1 && 0==V_ref && abs(V)>1 && 1==scPP) % Reset integral state and switch into braking mode
    % Conditions: velocity error large, velocity large, error and velocity
    % signs are different
    disp('Braking mode');
    state=0;
    scPP=1.8;
end

if (abs(DV)<1 && 1.8==scPP) % Switch back to normal mode
    % Condition: velocity error small
    disp('Back to normal mode');
    scPP=1;    
end

% control demand as integral state + proportional part
dmd = state + scPP*PP*DV;

% Test for saturation and AW
if (dmd > pitch_max)
    dmd = pitch_max; % Saturation
    if (DV > 0)      % continue integral if error sign acts away from the limit
        state = state + PI*DV*ts_hexacopter;
    end
elseif (dmd < -pitch_max)
    dmd = -pitch_max; % Saturation
    if (DV < 0)       % continue integral if error sign acts away from the limit
        state = state + PI*DV*ts_hexacopter;
    end
else % Integral of tracking error
    state = state + PI*DV*ts_hexacopter;
end

y = dmd;
end

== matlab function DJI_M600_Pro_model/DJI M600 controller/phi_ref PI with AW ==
function y  = fcn(V,V_ref,DV,RP,RI,ts_hexacopter,roll_max)
% PI control of roll angle with anti-windup (AW)
% Inputs:
% V:    actual velocity value
% DV:   velocity tracking error
% Parameters:
% RP:               roll proportional gain
% RI:               roll integral gain
% ts_hexacopter:    sampling time
% roll_max:        maximum allowed roll angle
% Output:
% dmd:  roll angle reference
%
% Institute for Computer Science and Control,  Budapest, Hungary
% Systems and Control Laboratory 2023.
% v3.0 12. June 2023.
%       

% State of integral control
persistent state
% RP gain scale in brake mode
persistent scPP

% Initialize persistent variables
if isempty(state)
    state = 0;
    % By default no brake scale
    scPP=1;
end

if (abs(DV)>1 && 0==V_ref && abs(V)>1 && 1==scPP) % Reset integral state and switch into braking mode
    % Conditions: velocity error large, velocity large, error and velocity
    % signs are different
    state=0;
    scPP=1.8;
end

if (abs(DV)<1 && 1.8==scPP) % Switch back to normal mode
    % Condition: velocity error small
    scPP=1;
end

% control demand as integral state + proportional part
dmd = state + scPP*RP*DV;

% Test for saturation and AW
if (dmd > roll_max)
    dmd = roll_max; % Saturation
    if (DV < 0)     % continue integral if error sign acts away from the limit
        state = state + RI*DV*ts_hexacopter;
    end
elseif (dmd < -roll_max)
    dmd = -roll_max; % Saturation
    if (DV > 0)      % continue integral if error sign acts away from the limit
        state = state + RI*DV*ts_hexacopter;
    end
else % Integral of tracking error
    state = state + RI*DV*ts_hexacopter;
end

y = dmd;
end

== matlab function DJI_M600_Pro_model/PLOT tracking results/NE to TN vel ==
function y = fcn(u)
% Transform North-East to Tangential-Normal
% Inputs
% u(1):     North position / velocity
% u(2):     East position / velocity
% u(3):     Real yaw angle
% Outputs
% T:    tangential position / velocity
% N:    normal position / velocity
%
% Institute for Computer Science and Control, Budapest, Hungary
% Systems and Control Laboratory 2023.
% v3.0 12. June 2023.

y = [u(1)*cos(u(3))+u(2)*sin(u(3)); -u(1)*sin(u(3))+u(2)*cos(u(3))];
